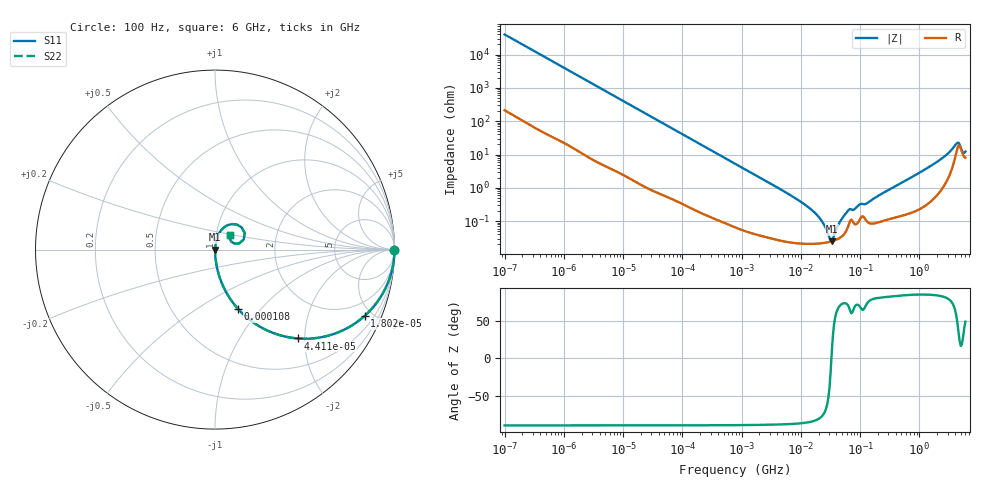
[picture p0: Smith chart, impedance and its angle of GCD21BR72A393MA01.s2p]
!Murata Part Number: GCD21BR72A393MA01
!These Parameters are Measured in Series Mode Connection
!Data Generated on Jan 08, 2026
!  o--ll--o
!Port1  Port2
!  o------o
!Operation Temp=25[degC], DC Bias Voltage=0[V]
!Freq. Start=100[Hz] Stop=6[GHz] 401[Steps]
# Hz S RI R 50
!Freq.(Hz) S11(Real) S11(Imag) S21(Real) S21(Imag) S12(Real) S12(Imag) S22(Real) S22(Imag)
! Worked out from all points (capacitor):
!   401 points, 100 Hz to 6 GHz, reference 50 ohm
!   read as one part in series: C = 39.8 nF near 109 Hz
!   lowest |Z| = 25.1 mohm at 33.3 MHz (marker M1)
!   series resonance near 32.87 MHz, so ESL is about 590 pH
!   S11 on the Smith chart (normalised r, x): 100 Hz: open; 18.02 kHz: 1.03, -4.52; 44.11 kHz: 1.01, -1.85; 108 kHz: 1.01, -0.76; 6 GHz: 1.16, +0.19
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100  1 -0.0025  1.96e-05 0.0025  1.96e-05 0.0025  1 -0.0025
2008  0.9973 -0.0496  0.00273 0.0496  0.00273 0.0496  0.9973 -0.0496
8047  0.9611 -0.1905  0.0389 0.1905  0.0389 0.1905  0.9611 -0.1905
18016  0.8346 -0.3685  0.1654 0.3685  0.1654 0.3685  0.8346 -0.3685
40335  0.5057 -0.4966  0.4943 0.4966  0.4943 0.4966  0.5057 -0.4966
44113  0.4615 -0.4951  0.5385 0.4951  0.5385 0.4951  0.4615 -0.4951
108014  0.1279 -0.3299  0.8721 0.3299  0.8721 0.3299  0.1279 -0.3299
276587  0.023 -0.1452  0.977 0.1452  0.977 0.1452  0.023 -0.1452
774597  0.00349 -0.0532  0.9965 0.0532  0.9965 0.0532  0.00349 -0.0532
6644369  0.000266 -0.00606  0.9997 0.00606  0.9997 0.00606  0.000266 -0.00606
1.555665e7  0.000213 -0.0021  0.9998 0.0021  0.9998 0.0021  0.000213 -0.0021
2.225763e7  0.000218 -0.00103  0.9998 0.00103  0.9998 0.00103  0.000218 -0.00103
3.045065e7  0.000239 -0.000198  0.9998 0.000198  0.9998 0.000198  0.000239 -0.000198
3.330331e7  0.000249 3.47e-05  0.9998 -3.47e-05  0.9998 -3.47e-05  0.000249 3.47e-05
4.556224e7  0.000317 0.000888  0.9997 -0.000888  0.9997 -0.000888  0.000317 0.000888
6.233367e7  0.000663 0.00194  0.9993 -0.00194  0.9993 -0.00194  0.000663 0.00194
1.334425e8  0.000961 0.00339  0.999 -0.00339  0.999 -0.00339  0.000961 0.00339
3.124326e8  0.00123 0.00883  0.9988 -0.00883  0.9988 -0.00883  0.00123 0.00883
1.873145e9  0.00833 0.055  0.9917 -0.055  0.9917 -0.055  0.00833 0.055
3.205649e9  0.0346 0.1083  0.9654 -0.1083  0.9654 -0.1083  0.0346 0.1083
4.193612e9  0.1205 0.1398  0.8795 -0.1398  0.8795 -0.1398  0.1205 0.1398
6e9  0.0812 0.079  0.9188 -0.079  0.9188 -0.079  0.0812 0.079
